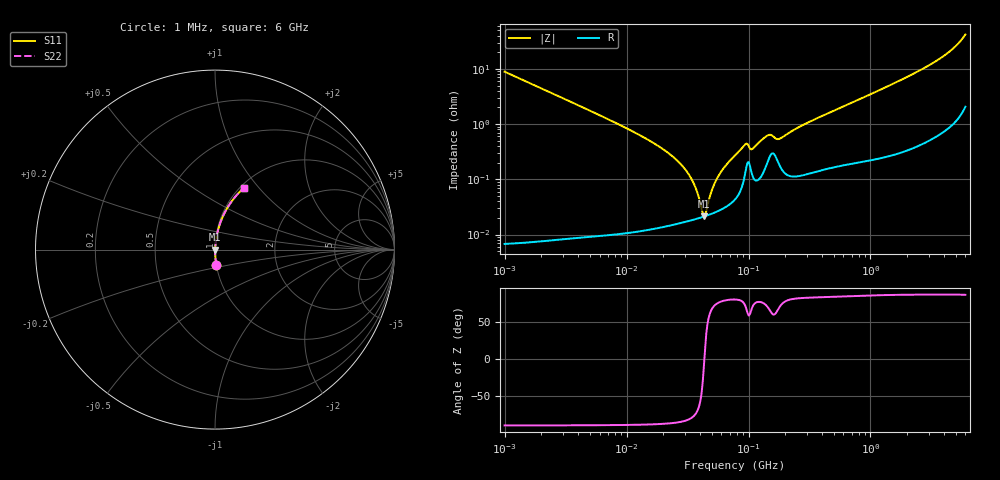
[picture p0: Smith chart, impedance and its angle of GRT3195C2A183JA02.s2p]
!Murata Part Number: GRT3195C2A183JA02
!These Parameters are Measured in Series Mode Connection
!Data Generated on Jun 19, 2026
!  o--ll--o
!Port1  Port2
!  o------o
!Operation Temp=25[degC], DC Bias Voltage=0[V]
!Freq. Start=1000[kHz] Stop=6[GHz] 401[Steps]
# Hz S RI R 50
!Freq.(Hz) S11(Real) S11(Imag) S21(Real) S21(Imag) S12(Real) S12(Imag) S22(Real) S22(Imag)
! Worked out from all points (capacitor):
!   401 points, 1 MHz to 6 GHz, reference 50 ohm
!   read as one part in series: C = 17.9 nF near 1.044 MHz
!   lowest |Z| = 21.4 mohm at 43.06 MHz (marker M1)
!   series resonance near 43.42 MHz, so ESL is about 750 pH
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1000000  0.00792 -0.0882  0.9921 0.0882  0.9921 0.0882  0.00792 -0.0882
4293785  0.000509 -0.0205  0.9995 0.0205  0.9995 0.0205  0.000509 -0.0205
1.843659e7  0.000148 -0.00394  0.9999 0.00394  0.9999 0.00394  0.000148 -0.00394
2.554826e7  0.00016 -0.00227  0.9998 0.00227  0.9998 0.00227  0.00016 -0.00227
3.175522e7  0.000176 -0.0013  0.9998 0.0013  0.9998 0.0013  0.000176 -0.0013
3.618157e7  0.000189 -0.000749  0.9998 0.000749  0.9998 0.000749  0.000189 -0.000749
4.12249e7  0.000205 -0.000212  0.9998 0.000212  0.9998 0.000212  0.000205 -0.000212
4.305766e7  0.000212 -3.39e-05  0.9998 3.39e-05  0.9998 3.39e-05  0.000212 -3.39e-05
4.497189e7  0.000219 0.000145  0.9998 -0.000145  0.9998 -0.000145  0.000219 0.000145
5.013812e7  0.000239 0.000596  0.9998 -0.000596  0.9998 -0.000596  0.000239 0.000596
5.589783e7  0.000266 0.00106  0.9997 -0.00106  0.9997 -0.00106  0.000266 0.00106
6.368941e7  0.000309 0.00165  0.9997 -0.00165  0.9997 -0.00165  0.000309 0.00165
7.745967e7  0.000438 0.00268  0.9996 -0.00268  0.9996 -0.00268  0.000438 0.00268
9.420718e7  0.00134 0.0041  0.9987 -0.0041  0.9987 -0.0041  0.00134 0.0041
1.073387e8  0.0012 0.00333  0.9988 -0.00333  0.9988 -0.00333  0.0012 0.00333
1.455431e8  0.00228 0.00589  0.9977 -0.00589  0.9977 -0.00589  0.00228 0.00589
1.809028e8  0.00176 0.00516  0.9982 -0.00516  0.9982 -0.00516  0.00176 0.00516
3.325952e8  0.00144 0.0115  0.9986 -0.0115  0.9986 -0.0115  0.00144 0.0115
1.428092e9  0.0051 0.0496  0.9949 -0.0496  0.9949 -0.0496  0.0051 0.0496
3.5601e9  0.0263 0.1402  0.9737 -0.1402  0.9737 -0.1402  0.0263 0.1402
4.93336e9  0.0683 0.2317  0.9317 -0.2317  0.9317 -0.2317  0.0683 0.2317
6e9  0.1619 0.3445  0.8381 -0.3445  0.8381 -0.3445  0.1619 0.3445
